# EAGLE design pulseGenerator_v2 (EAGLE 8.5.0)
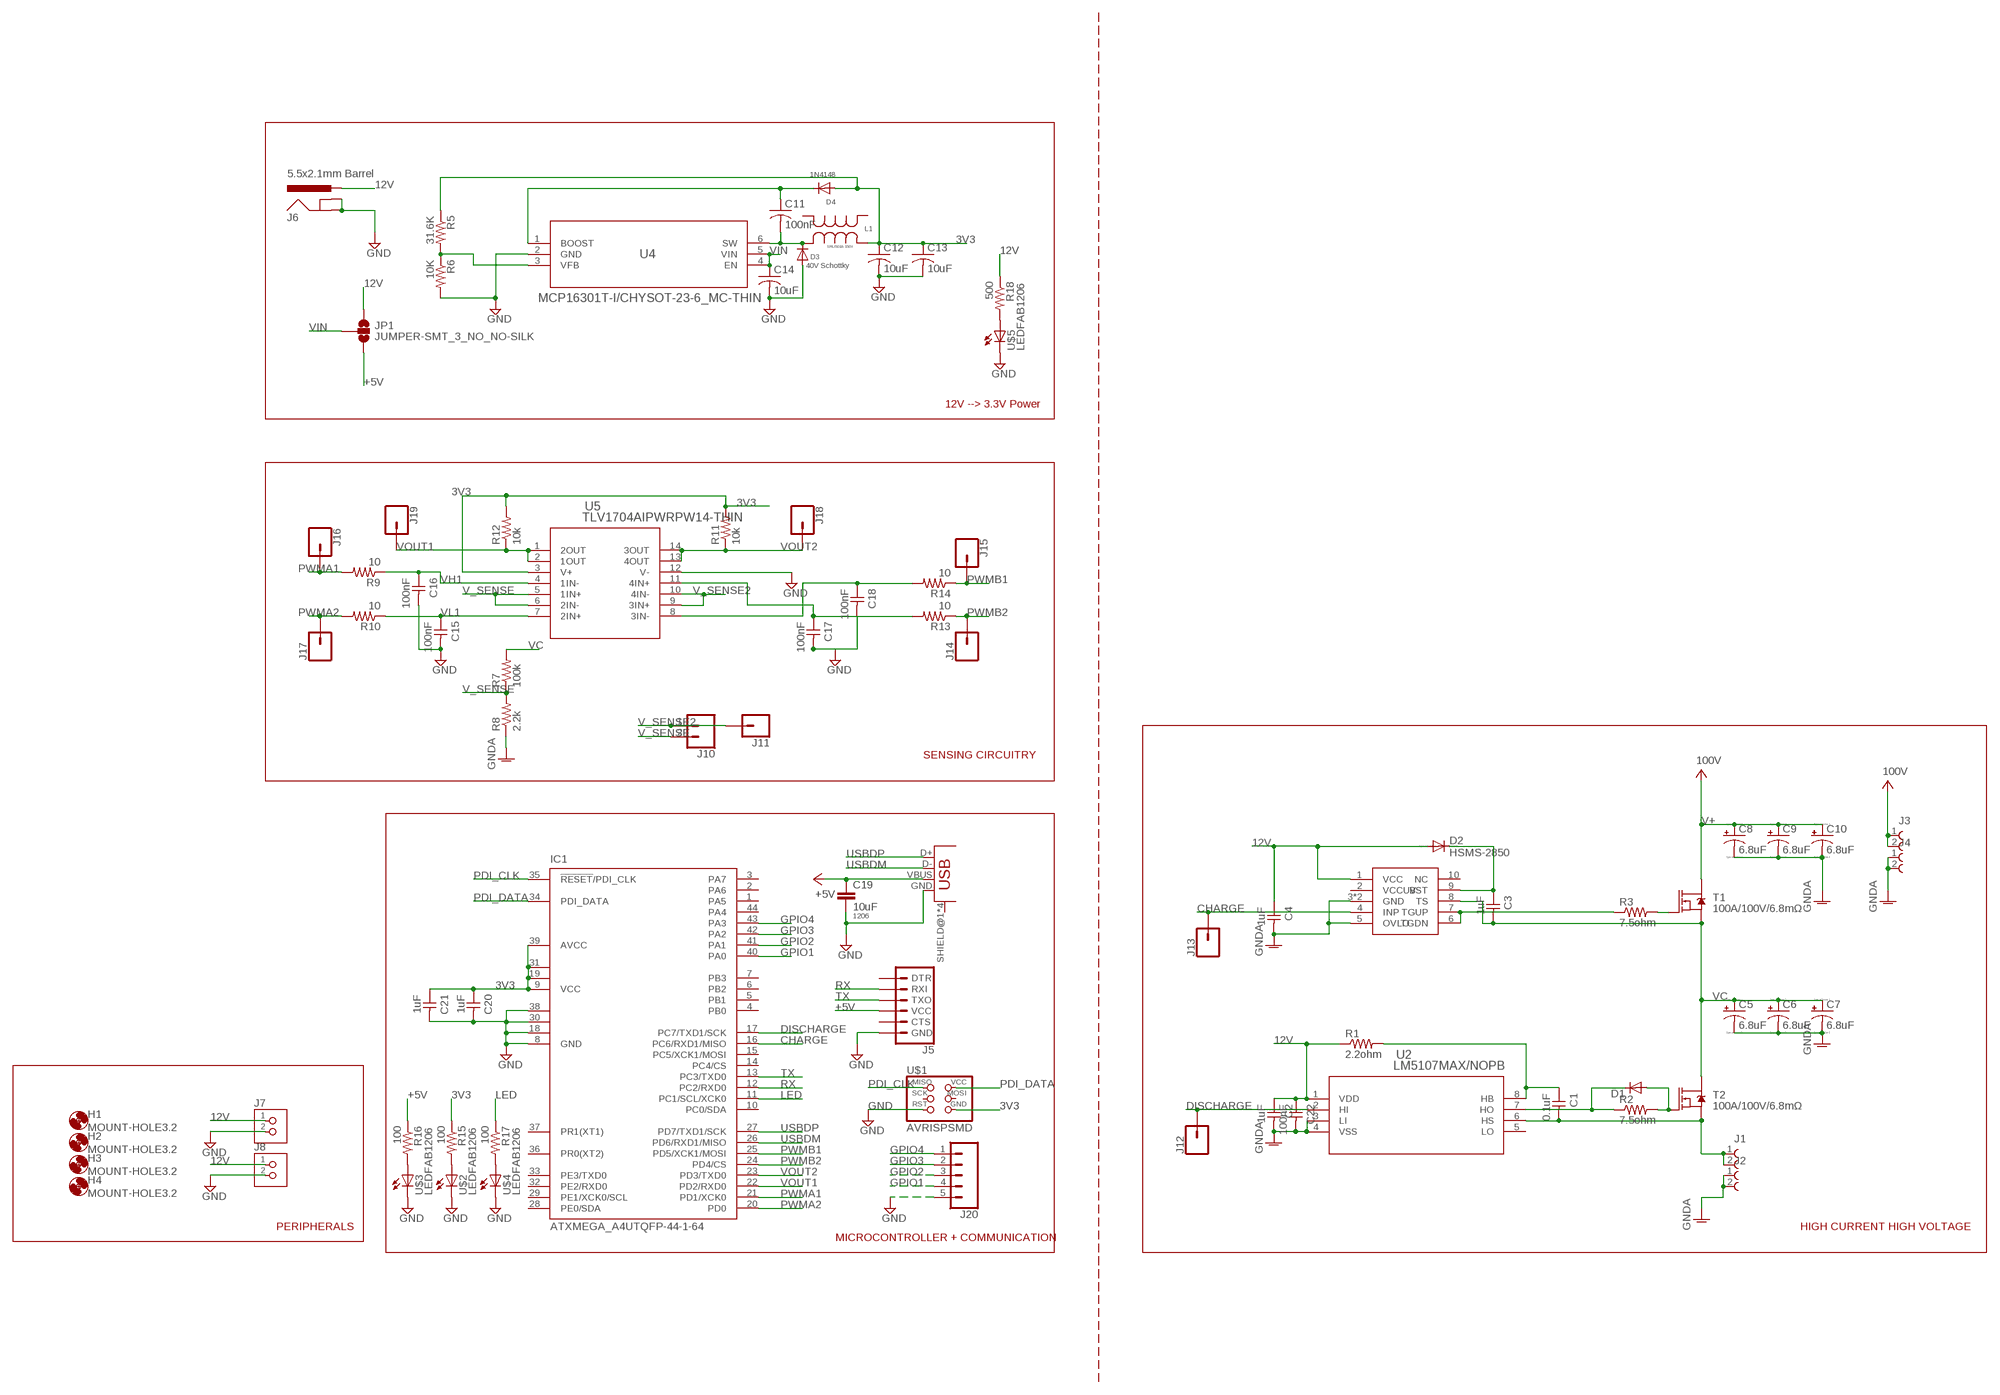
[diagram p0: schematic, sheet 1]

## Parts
C1  0.1uF  CAP-UNPOLARIZEDFAB  [C1206FAB]
C2  1uF  CAP-UNPOLARIZEDFAB  [C1206FAB]
C3  1uF  CAP-UNPOLARIZEDFAB  [C1206FAB]
C4  1uF  CAP-UNPOLARIZEDFAB  [C1206FAB]
C5  6.8uF  CPOL-USF  [PANASONIC_F]
C6  6.8uF  CPOL-USF  [PANASONIC_F]
C7  6.8uF  CPOL-USF  [PANASONIC_F]
C8  6.8uF  CPOL-USF  [PANASONIC_F]
C9  6.8uF  CPOL-USF  [PANASONIC_F]
C10  6.8uF  CPOL-USF  [PANASONIC_F]
C11  100nF  C-USC1206  [C1206]
C12  10uF  C-USC1206  [C1206]
C13  10uF  C-USC1206  [C1206]
C14  10uF  C-USC1206  [C1206]
C15  100nF  CAP-UNPOLARIZEDFAB  [C1206FAB]
C16  100nF  CAP-UNPOLARIZEDFAB  [C1206FAB]
C17  100nF  CAP-UNPOLARIZEDFAB  [C1206FAB]
C18  100nF  CAP-UNPOLARIZEDFAB  [C1206FAB]
C19  10uF  CAP1206  [1206]
C20  1uF  CAP-UNPOLARIZEDFAB  [C1206FAB]
C21  1uF  CAP-UNPOLARIZEDFAB  [C1206FAB]
C22  100nF  CAP-UNPOLARIZEDFAB  [C1206FAB]
D1  DIODESOD123  [SOD123]
D2  HSMS-2850  [SOT23]
D3  40V Schottky  DIODESOD-123  [SOD-123]
D4  1N4148  DIODESOD-123  [SOD-123]
H1  MOUNT-HOLE3.2  [3,2]
H2  MOUNT-HOLE3.2  [3,2]
H3  MOUNT-HOLE3.2  [3,2]
H4  MOUNT-HOLE3.2  [3,2]
IC1  ATXMEGA_A4UTQFP-44-1-64  [TQFP44-13THIN]
J1  691236510002  [691236510002]
J2  691236510002  [691236510002]
J3  691236510002  [691236510002]
J4  691236510002  [691236510002]
J5  6_PIN_SERIAL_TARGETRA_SMT  [6_PIN_SERIAL_TARGET_SIDE_RA_SMT]
J6  5.5x2.1mm Barrel  POWER_JACKSMD  [POWER_JACK_SMD]
J7  TERM-1X02-FABLAB  [ED555DS-2DS]
J8  TERM-1X02-FABLAB  [ED555DS-2DS]
J10  CONN_02  [1X02]
J11  CONN_01  [1X01]
J12  CONN_01  [1X01]
J13  CONN_01  [1X01]
J14  CONN_01  [1X01]
J15  CONN_01  [1X01]
J16  CONN_01  [1X01]
J17  CONN_01  [1X01]
J18  CONN_01  [1X01]
J19  CONN_01  [1X01]
J20  CONN_05  [1X05]
JP1  JUMPER-SMT_3_NO_NO-SILK  [SMT-JUMPER_3_NO_NO-SILK]
L1  SRU5018-150Y  [IND_BOURNS_SRU5018]
R1  2.2ohm  R-US_R1206  [R1206]
R2  7.5ohm  R-US_R1206  [R1206]
R3  7.5ohm  R-US_R1206  [R1206]
R5  31.6K  RES-US1206FAB  [R1206FAB]
R6  10K  R-US_R1206  [R1206]
R7  100k  R-US_R1206  [R1206]
R8  2.2k  R-US_R1206  [R1206]
R9  10  RES-US1206FAB  [R1206FAB]
R10  10  RES-US1206FAB  [R1206FAB]
R11  10k  RES-US1206FAB  [R1206FAB]
R12  10k  RES-US1206FAB  [R1206FAB]
R13  10  RES-US1206FAB  [R1206FAB]
R14  10  RES-US1206FAB  [R1206FAB]
R15  100  R-US_R1206  [R1206]
R16  100  R-US_R1206  [R1206]
R17  100  R-US_R1206  [R1206]
R18  500  R-US_R1206  [R1206]
T1  100A/100V/6.8mΩ  MOSFET-NCH-PSMN7R0  [TO-263/D2PAK]
T2  100A/100V/6.8mΩ  MOSFET-NCH-PSMN7R0  [TO-263/D2PAK]
U2  LM5107MAX/NOPB  [M08A]
U4  MCP16301T-I/CHYSOT-23-6_MC-THIN  [SOT-23-6_MC-THIN]
U5  TLV1704AIPWRPW14-THIN  [PW14_THIN]
U$1  AVRISPSMD  [2X03SMD]
U$2  LEDFAB1206  [LED1206FAB]
U$3  LEDFAB1206  [LED1206FAB]
U$4  LEDFAB1206  [LED1206FAB]
U$5  LEDFAB1206  [LED1206FAB]
U$6  LTC7001  [LTC7001-10MSOP]
X1  USB_MINIB  [USB_MINIB]

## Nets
3V3 [signal]: C12.1 C13.1 C20.1 C21.1 D4.A IC1.9(VCC) IC1.19(VCC1) IC1.31(VCC2) IC1.39(AVCC) L1.1 R5.1 R11.2 R12.2 R15.1 U5.3(V+) U$1.6(GND)
12V [signal]: C2.1 C4.1 C22.1 D2.1(A) J6.VIN0(PWR) J7.1 J8.1 JP1.1 R1.1 R18.1 U2.1(VDD) U$6.1(VCC)
+5V: C19.1 J5.4(VCC) JP1.3 R16.1 X1.VBUS
CHARGE [signal]: IC1.16(PC6/RXD1/MISO) J13.1 U$6.4(INP)
DISCHARGE [signal]: IC1.17(PC7/TXD1/SCK) J12.1 U2.2(HI)
GND: C12.2 C13.2 C14.2 C15.2 C16.2 C17.2 C18.2 C19.2 C20.2 C21.2 D3.A IC1.8(GND) IC1.18(GND1) IC1.30(GND2) IC1.38(GND3) J5.6(GND) J6.GND(GNDBREAK) J6.P$4(GND) J7.2 J8.2 J20.5 R6.2 U4.2(GND) U5.12(V-) U$1.5(RST) U$2.2(C) U$3.2(C) U$4.2(C) U$5.2(C) X1.GND
GNDA [POWER]: C2.2 C4.2 C5.- C6.- C7.- C8.- C9.- C10.- C22.2 J2.1 J2.2 J4.1 J4.2 R8.1 U2.3(LI) U2.4(VSS) U$6.3(GND) U$6.5(OVLO) U$6.P$1(GND)
GPIO1: IC1.40(PA0) J20.4
GPIO2: IC1.41(PA1) J20.3
GPIO3: IC1.42(PA2) J20.2
GPIO4: IC1.43(PA3) J20.1
LED [signal]: IC1.11(PC1/SCL/XCK0) R17.1
N$1 [signal]: C3.1 D2.3(C) U$6.9(BST)
N$2 [signal]: C1.1 R1.2 U2.8(HB)
N$3: R15.2 U$2.1(A)
N$4 [signal]: D1.ANODE(A) R2.2 T2.1(G)
N$5 [signal]: D1.CATHODE(C) R2.1 U2.7(HO)
N$6: R16.2 U$3.1(A)
N$9: R3.2 T1.1(G)
N$10 [signal]: R3.1 U$6.6(TGDN) U$6.7(TGUP)
N$11 [signal]: C17.1 R13.2 U5.11(4IN+)
N$12: R17.2 U$4.1(A)
N$13 [signal]: C11.2 D3.C L1.3 U4.6(SW)
N$14: R18.2 U$5.1(A)
N$15 [signal]: C11.1 D4.C U4.1(BOOST)
N$18 [signal]: C18.1 R14.2 U5.8(3IN-)
N$19 [signal]: R5.2 R6.1 U4.3(VFB)
OUTPUT [POWER]: C1.2 J1.1 J1.2 T2.3(S) U2.6(HS)
PDI_CLK [signal]: IC1.35(!RESET!/PDI_CLK) U$1.1(MISO)
PDI_DATA [signal]: IC1.34(PDI_DATA) U$1.2(VCC)
PWMA1 [signal]: IC1.21(PD1/XCK0) J16.1 R9.2
PWMA2 [signal]: IC1.20(PD0) J17.1 R10.2
PWMB1 [signal]: IC1.25(PD5/XCK1/MOSI) J15.1 R14.1
PWMB2 [signal]: IC1.24(PD4/CS) J14.1 R13.1
RX [signal]: IC1.12(PC2/RXD0) J5.3(RXI)
TX [signal]: IC1.13(PC3/TXD0) J5.2(TXO)
USBDM [signal]: IC1.26(PD6/RXD1/MISO) X1.D-
USBDP [signal]: IC1.27(PD7/TXD1/SCK) X1.D+
V+ [POWER]: C8.+ C9.+ C10.+ J3.1 J3.2 T1.2(D) ; supply symbol labelled 100V
V_SENSE [signal]: J10.2 R7.1 R8.2 U5.5(1IN+) U5.6(2IN-)
V_SENSE2 [signal]: J10.1 J11.1 U5.9(3IN+) U5.10(4IN-)
VC [signal]: C3.2 C5.+ C6.+ C7.+ R7.2 T1.3(S) T2.2(D) U$6.8(TS)
VH1 [signal]: C16.1 R9.1 U5.4(1IN-)
VIN: C14.1 JP1.2 U4.4(EN) U4.5(VIN)
VL1 [signal]: C15.1 R10.1 U5.7(2IN+)
VOUT1 [signal]: IC1.22(PD2/RXD0) J19.1 R12.1 U5.1(2OUT) U5.2(1OUT)
VOUT2 [signal]: IC1.23(PD3/TXD0) J18.1 R11.1 U5.13(4OUT) U5.14(3OUT)
Unconnected: IC1.1(PA5) IC1.2(PA6) IC1.3(PA7) IC1.4(PB0) IC1.5(PB1) IC1.6(PB2) IC1.7(PB3) IC1.10(PC0/SDA) IC1.14(PC4/CS) IC1.15(PC5/XCK1/MOSI) IC1.28(PE0/SDA) IC1.29(PE1/XCK0/SCL) IC1.32(PE2/RXD0) IC1.33(PE3/TXD0) IC1.36(PR0(XT2)) IC1.37(PR1(XT1)) IC1.44(PA4) J5.1(DTR) J5.5(CTS) L1.2 L1.4 U2.5(LO) U$1.3(SCK) U$1.4(MOSI) U$6.2(VCCUV) U$6.10(NC) X1.SHIELD@1(SHIELD) X1.SHIELD@2(SHIELD) X1.SHIELD@3(SHIELD) X1.SHIELD@4(SHIELD)

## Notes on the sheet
- 12V --> 3.3V Power
- SENSING CIRCUITRY
- PERIPHERALS | HIGH CURRENT HIGH VOLTAGE
- MICROCONTROLLER + COMMUNICATION

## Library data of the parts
C1-C4 C15-C18 C20-C22 = fab:CAP-UNPOLARIZED
C5-C10 = resistor:CPOL-US: POLARIZED CAPACITOR, American symbol
C11-C14 = resistor:C-US: CAPACITOR, American symbol
C19 = borkedlabs-passives:CAP: Capacitor; PACKAGE: 1206
D1 = fab:DIODE: DIODE
D2 = avago:HSMS-2850: Surface Mount Microwave Schottky Detector Diodes
D3 D4 = adafruit:DIODE: Diode
H1-H4 = holes:MOUNT-HOLE: MOUNTING HOLE with drill center marker
IC1 = fab:ATXMEGA_A4U
J1-J4 = Wurth_Elektronik_Electromechanic_Terminal_Blocks_Connectors_rev17a:691236510002
J5 = SparkFun-Connectors:6_PIN_SERIAL_TARGET: 6-pin header connection for use with the "FTDI BASIC" pinout - TARGET SIDE. Also known as "Arduino Serial Program Header". It is used to mate with our FTDI Basic serial programmers using the Arduino IDE. Note, this device has "TARGET" in the name. It is intended to be used on a design that contains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; PROD_ID: CONN-08971
J6 = SparkFun-Connectors:POWER_JACK: Power Jack Connector This is the standard 5.5mm barrel jack for power. The PTH is the most common, proven, reliable, footprint. The Slot footprint only works if the mill layer is transmitted to the PCB fab house so be warned. Here are the connectors we sell at SparkFun: DC Barrel Power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; PROD_ID: CONN-08106; SF_ID: PRT-12748
J7 J8 = fab:TERM-1X02: 3.5mm terminal block, 2 positions ED555-2DS as found in the fablab inventory.
J10 = SparkFun-Connectors:CONN_02: Multi connection point. Often used as Generic Header-pin footprint for 0.1 inch spaced/style header connections
J11-J19 = SparkFun-Connectors:CONN_01: Single connection point. Often used as Generic Header-pin footprint for 0.1 inch spaced/style header connections
J20 = SparkFun-Connectors:CONN_05: Multi connection point. Often used as Generic Header-pin footprint for 0.1 inch spaced/style header connections On any of the 0.1 inch spaced packages, you can populate with these: Break Away Headers - Straight (PRT-00116) Break Away Male Headers - Right Angle (PRT-00553) Female Headers (PRT-00115)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
JP1 = SparkFun-Jumpers:JUMPER-SMT_3_NO: Normally open jumper This jumper has three pads in close proximity to each other. Apply solder to close the connection(s).
L1 = will:SRU5018-150Y; MANUFACTURER_PART_NUMBER: SRU5018150Y; VENDOR: Bourns Electronics
R1-R3 R6-R8 R15-R18 = resistor:R-US_: RESISTOR, American symbol
R5 R9-R14 = fab:RES-US: Resistor (US Symbol)
T1 T2 = SparkFun-DiscreteSemi:MOSFET-NCH: N-channel MOSFETs Voltage controlled devices that allow control of high current outputs. SparkFun Products: SparkFun OpenScale SparkFun Digital Sandbox SparkFun Monster Moto Shield SparkFun MOSFET Power Controller; PROD_ID: TRANS-12437
U2 = lm5107_half_bridge_gate_driver:LM5107MAX/NOPB; MANUFACTURER_PART_NUMBER: LM5107MAXNOPB; VENDOR: Texas Instruments
U4 = will:MCP16301T-I/CHY
U5 = will:TLV1704AIPWR
U$1 = fab:AVRISP
U$2-U$5 = fab:LED: LED
U$6 = will:LTC7001
X1 = fab:USB_MINIB

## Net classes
0 default: width 0.305 mm, clearance 0.45 mm
1 POWER: width 1.27 mm, clearance 2 mm
2 signal: width 0.25 mm, clearance 0.2 mm

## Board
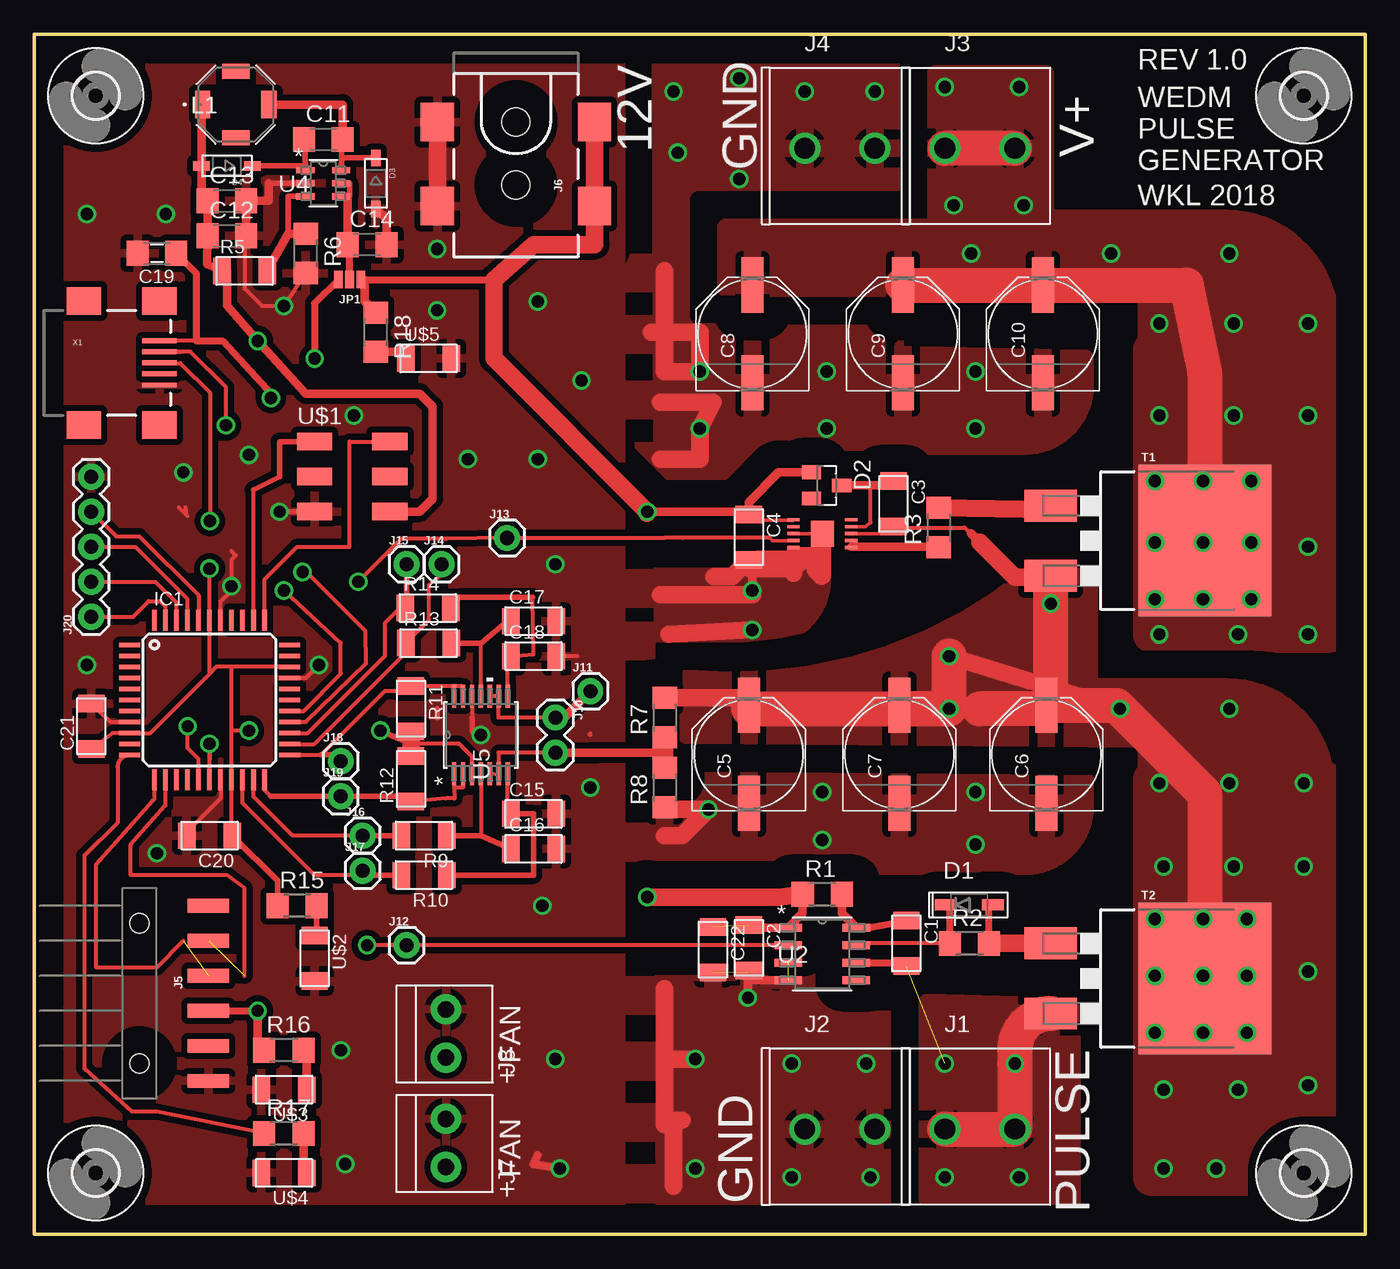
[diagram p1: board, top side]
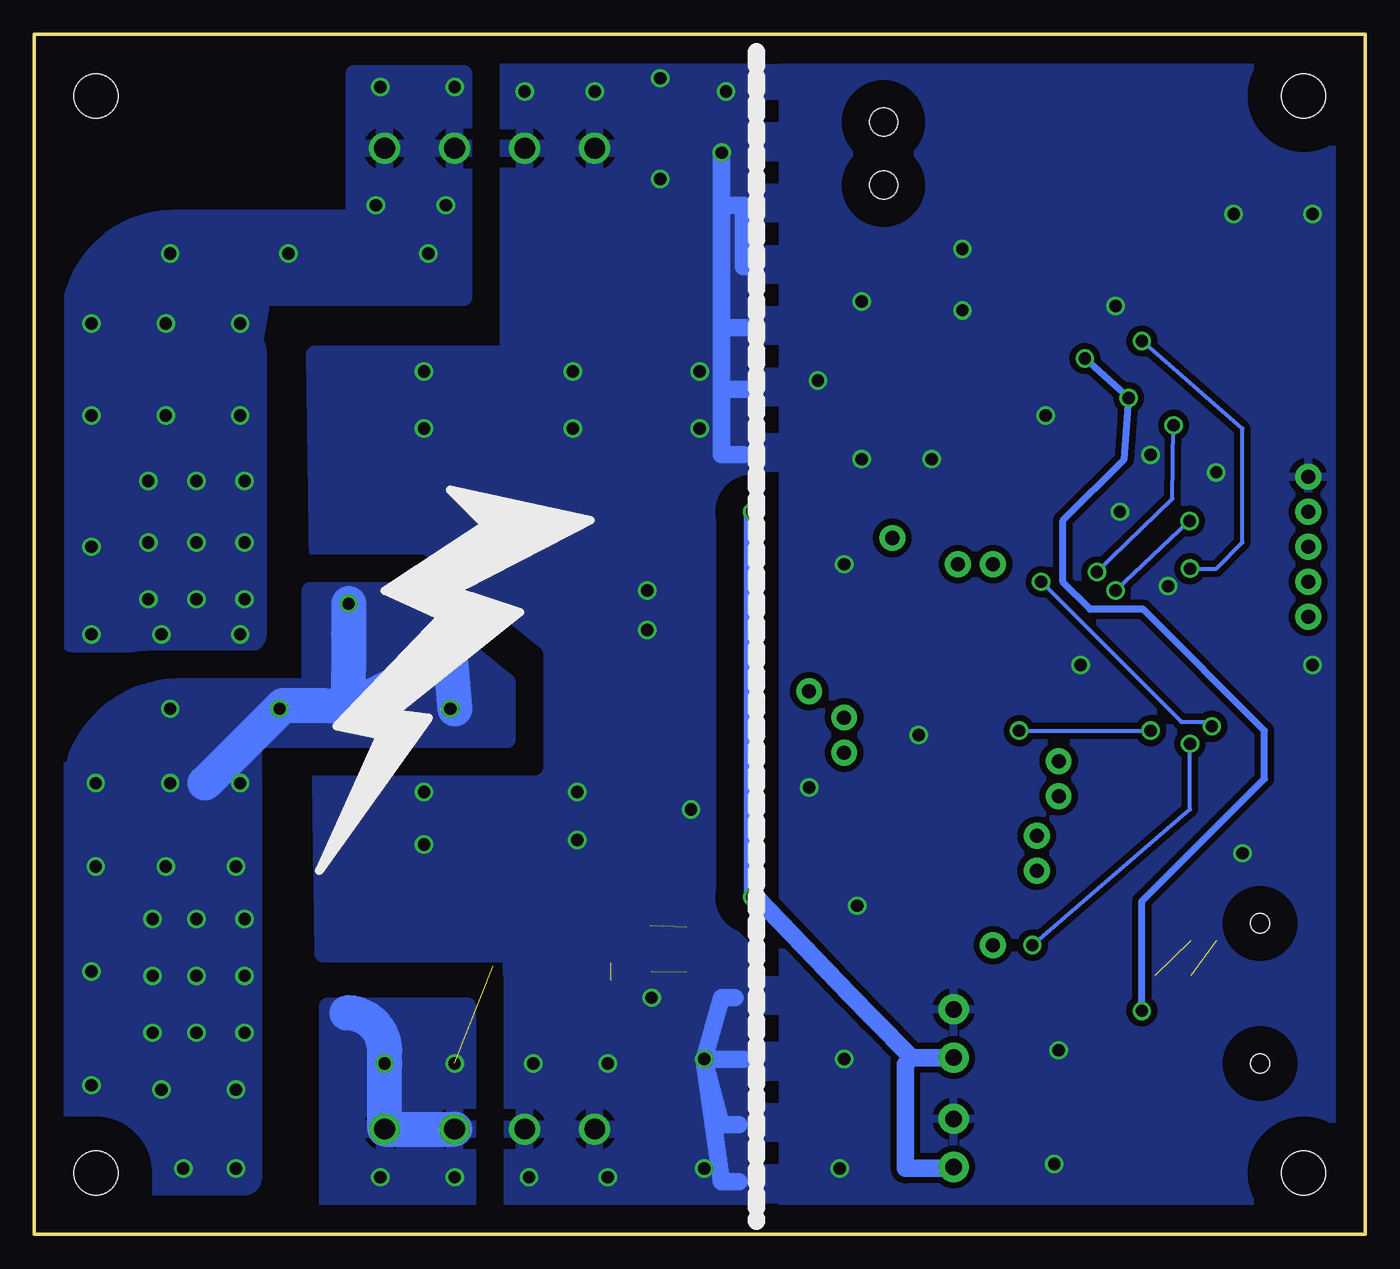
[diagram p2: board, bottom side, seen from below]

Size 96.52 x 87 mm. Coordinates in mm from the lower left corner, seen from the top.
Outline: 0,0 96.52,0 96.52,87 0,87 0,0
Copper layers (1*16): Top 0.035mm / dielectric 1.5mm / Bottom 0.035mm
Design rules "default *": minimum track width 6mil, minimum drill 0.35mm, track to track 0.2mm, track to pad 0.2mm, pad to pad 0.2mm, via to via 0.2mm, smd to smd 0mil, copper to edge 2mm, drill to drill 6mil, minimum pad ring 10mil, minimum via ring 8mil, stop-mask expansion 4mil, vias tented up to drill 0mil, thermal gap 0.45mm

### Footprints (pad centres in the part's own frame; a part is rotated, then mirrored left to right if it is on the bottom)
C1206FAB = smd 1.27 x 1.905: 1 -1.651,0; 2 1.651,0
PANASONIC_F = smd 4 x 1.6: + 3.55,0; - -3.55,0
C1206 = smd 1.6 x 1.8: 1 -1.4,0; 2 1.4,0
1206 = smd 1.6 x 1.8: 1 -1.4,0; 2 1.4,0
SOD123 = smd 1.6 x 0.8: ANODE 1.7,0; CATHODE -1.7,0
SOT23 = smd 1 x 1.4: 1 -0.95,-1.1; 2 0.95,-1.1; 3 0,1.1
SOD-123 = smd 1.2 x 0.7: A 1.85,0; C -1.85,0
3,2 = hole 3.2: 0,0
TQFP44-13THIN = smd 1.524 x 0.33: 1 -5.8,4; 2 -5.8,3.2; 3 -5.8,2.4; 4 -5.8,1.6; 5 -5.8,0.8; 6 -5.8,0; 7 -5.8,-0.8; 8 -5.8,-1.6; 9 -5.8,-2.4; 10 -5.8,-3.2; 11 -5.8,-4; 23 5.8,-4; 24 5.8,-3.2; 25 5.8,-2.4; 26 5.8,-1.6; 27 5.8,-0.8; 28 5.8,0; 29 5.8,0.8; 30 5.8,1.6; 31 5.8,2.4; 32 5.8,3.2; 33 5.8,4 | smd 0.33 x 1.524: 12 -4,-5.8; 13 -3.2,-5.8; 14 -2.4,-5.8; 15 -1.6,-5.8; 16 -0.8,-5.8; 17 0,-5.8; 18 0.8,-5.8; 19 1.6,-5.8; 20 2.4,-5.8; 21 3.2,-5.8; 22 4,-5.8; 34 4,5.8; 35 3.2,5.8; 36 2.4,5.8; 37 1.6,5.8; 38 0.8,5.8; 39 0,5.8; 40 -0.8,5.8; 41 -1.6,5.8; 42 -2.4,5.8; 43 -3.2,5.8; 44 -4,5.8
691236510002 = drill 1.5: 1 -2.54,0; 2 2.54,0
6_PIN_SERIAL_TARGET_SIDE_RA_SMT = smd 1 x 3: 1 -6.35,5; 2 -3.81,5; 3 -1.27,5; 4 1.27,5; 5 3.81,5; 6 6.35,5 | hole 1.4: -5.08,0; 5.08,0
POWER_JACK_SMD = smd 2.8 x 2.4: GND 0,-5.7; P$4 6.1,-5.7; VIN0 0,5.7; VIN1 6.1,5.7 | hole 2.032: 0,0; 4.572,0
ED555DS-2DS = drill 1.2 pad 2.184: 1 1.8,0; 2 -1.7,0
1X02 = drill 1.016 pad 1.88: 1 0,0; 2 2.54,0
1X01 = drill 1.016 pad 1.88: 1 0,0
1X05 = drill 1.016 pad 1.88: 1 0,0; 2 2.54,0; 3 5.08,0; 4 7.62,0; 5 10.16,0
SMT-JUMPER_3_NO_NO-SILK = smd 0.635 x 1.27: 1 -0.813,0; 2 0,0; 3 0.813,0
IND_BOURNS_SRU5018 = smd 1.092 x 2.007: 1 -2.4,0; 3 2.4,0 | smd 2.007 x 1.092: 2 0,-2.4; 4 0,2.4
R1206 = smd 1.6 x 1.803: 1 -1.422,0; 2 1.422,0
R1206FAB = smd 1.27 x 1.905: 1 -1.651,0; 2 1.651,0
TO-263/D2PAK = smd 2.32 x 3.81: 1 -2.54,-7.045; 3 2.54,-7.045 | smd 11 x 9.65: 2 0,4.125
M08A = smd 1.981 x 0.559: 1 -2.464,1.905; 2 -2.464,0.635; 3 -2.464,-0.635; 4 -2.464,-1.905; 5 2.464,-1.905; 6 2.464,-0.635; 7 2.464,0.635; 8 2.464,1.905
SOT-23-6_MC-THIN = smd 1.321 x 0.457: 1 -1.295,0.95; 2 -1.295,0; 3 -1.295,-0.95; 4 1.295,-0.95; 5 1.295,0; 6 1.295,0.95
PW14_THIN = smd 1.676 x 0.305: 1 -2.819,1.95; 2 -2.819,1.3; 3 -2.819,0.65; 4 -2.819,0; 5 -2.819,-0.65; 6 -2.819,-1.3; 7 -2.819,-1.95; 8 2.819,-1.95; 9 2.819,-1.3; 10 2.819,-0.65; 11 2.819,0; 12 2.819,0.65; 13 2.819,1.3; 14 2.819,1.95
2X03SMD = smd 2.54 x 1.27: 1 -2.54,2.54; 2 2.92,2.54; 3 -2.54,0; 4 2.92,0; 5 -2.54,-2.54; 6 2.92,-2.54
LED1206FAB = smd 1.27 x 1.905: 1 -1.651,0; 2 1.651,0
LTC7001-10MSOP = smd 0.24 x 0.889: 1 -1,-2.1; 2 -0.5,-2.1; 3 0,-2.1; 4 0.5,-2.1; 5 1,-2.1; 6 1,2.1; 7 0.5,2.1; 8 0,2.1; 9 -0.5,2.1; 10 -1,2.1 | smd 1.88 x 1.68: P$1 0,0
USB_MINIB = smd 2.5 x 0.35: D+ 3.77,0; D- 3.77,0.8; GND 3.77,-1.6; ID 3.77,-0.8; VBUS 3.77,1.6 | smd 2.5 x 2: SHIELD@1 -1.73,-4.5; SHIELD@2 -1.73,4.5; SHIELD@3 3.77,4.5; SHIELD@4 3.77,-4.5

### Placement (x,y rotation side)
C1  63.25,21.08 270 top
C2  51.82,20.76 270 top
C3  62.32,52.96 270 top
C4  51.82,50.55 270 top
C5  51.82,34.8 90 top
C6  73.41,34.8 90 top
C7  62.74,34.8 90 top
C8  52.07,65.28 90 top
C9  62.99,65.28 90 top
C10  73.15,65.28 90 top
C11  20.95,79.38 0 top
C12  13.97,72.39 0 top
C13  13.97,74.93 0 top
C14  24.13,71.75 0 top
C15  36.2,30.48 0 top
C16  36.2,27.94 0 top
C17  36.2,44.45 0 top
C18  36.2,41.91 0 top
C19  8.89,71.12 180 top
C20  12.7,28.89 180 top
C21  4.13,36.83 90 top
C22  49.21,20.64 270 top
D1  67.82,23.88 0 top
D2  57.47,54.29 270 top
D3  24.77,76.2 270 top
D4  13.97,77.47 180 top
H1  4.45,4.45 0 top
H2  92.08,82.55 0 top
H3  4.45,82.55 0 top
H4  92.08,4.45 0 top
IC1  12.7,38.73 0 top
J1  68.58,7.62 0 top
J2  58.42,7.62 0 top
J3  68.58,78.74 0 top
J4  58.42,78.74 0 top
J5  7.62,17.46 270 top
J6  34.92,80.64 270 top
J7  29.84,6.67 270 top
J8  29.84,14.61 270 top
J10  37.78,37.47 270 top
J11  40.32,39.37 0 top
J12  26.99,20.95 0 top
J13  34.29,50.48 0 top
J14  29.53,48.58 0 top
J15  26.99,48.58 0 top
J16  23.81,28.89 0 top
J17  23.81,26.35 0 top
J18  22.23,34.29 0 top
J19  22.23,31.75 0 top
J20  4.13,44.77 90 top
JP1  22.86,69.22 180 top
L1  14.61,81.92 0 top
R1  57.15,24.64 0 top
R2  67.82,21.08 0 top
R3  65.6,51.24 90 top
R5  15.24,69.85 0 top
R6  19.68,71.12 270 top
R7  45.72,37.47 90 top
R8  45.72,32.38 90 top
R9  28.26,28.89 180 top
R10  28.26,26.04 180 top
R11  27.3,38.1 270 top
R12  27.3,33.02 90 top
R13  28.57,42.86 0 top
R14  28.55,45.4 0 top
R15  19.05,23.81 0 top
R16  18.1,13.34 0 top
R17  18.1,7.3 0 top
R18  24.77,65.41 270 top
T1  80.77,50.29 270 top
T2  80.77,18.54 270 top
U2  57.15,20.32 0 top
U4  20.95,76.2 0 top
U5  32.38,36.2 90 top
U$1  22.86,54.93 0 top
U$2  20.32,20 270 top
U$3  18.1,10.48 180 top
U$4  18.1,4.45 180 top
U$5  28.57,63.5 0 top
U$6  57.15,50.8 270 top
X1  5.31,63.18 0 top

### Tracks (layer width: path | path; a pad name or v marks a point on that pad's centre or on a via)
3V3  (via drill 0.89)
  Top 0.305: 31.75,33.31 arc90 U5.3 31.73,34.61 30.79,35.56 27.3,35.56 | IC1.19 14.3,29.09 C20.1 | IC1.19 | C21.1 5.67,36.34 IC1.9 8.39,36.34 12.7,40.64 | 12.7,40.64 IC1.39 v12.7,48.26 | IC1.31 14.29,41.13 | 14.29,41.13 13.2,41.13 12.7,40.64 | 14.29,36.51 14.29,32.95 IC1.19 | 14.29,36.51 14.29,41.13 | v15.56,36.51 14.29,36.51 | IC1.19
  Top 0.406: 27.3,35.56 v25.08,36.51 | R15.1 17.63,25.61 C20.1
  Top 0.61: 12.12,82.55 D4.A 12.12,74.93 C13.1 C12.1 12.54,70.33 R5.1 13.97,69.85 13.97,67.31 v16.19,64.77 19.68,60.96 27.94,60.96 28.89,60.01 28.89,53.34 27.94,52.39 U$1.6 | 12.12,82.55 12.06,81.92 | 12.12,82.55 12.21,82.55 L1.1
  Top 1.27: R12.2 27.3,35.56 R11.2
  Bottom 0.305: v25.08,36.51 v15.56,36.51 | v12.7,48.26 10.79,48.26 8.89,50.16 8.89,58.42 v16.19,64.77
12V  (via drill 0.89)  (1 unrouted)
  Top 0.241: U$6.1 55.05,51.75 51.82,51.75 C4.1
  Top 0.508: JP1.1 23.93,69.22 33.34,69.22
  Top 0.61: R1.1 55.73,23.27 U2.1 52.07,22.23 C2.1 | R18.1 23.93,67.66 23.93,69.22 | D2.1 53.97,55.24 51.82,53.09 C4.1 51.63,52.39 v44.45,52.39
  Top 1.27: J6.VIN0 40.64,80.63 40.64,71.75 36.2,71.75 33.34,69.22 33.34,63.5 v44.45,52.39 44.45,52.26 | R1.1 54.01,24.45 v44.45,24.45
  Bottom 1.27: v44.45,52.39 v44.45,24.45 44.13,24.45 37.31,17.31 35.79,15.72 32.87,12.8 | J8.1 32.87,12.8 | J7.1 29.95,4.76 33.34,4.76 33.34,12.34 32.87,12.8
+5V  (via drill 0.89)
  Top 0.305: X1.VBUS 9.84,64.78 | 9.84,64.78 10.3,64.78 | 11.75,64.77 11.73,64.78 9.84,64.78
  Top 0.508: JP1.3 20.32,67.49 v20.32,63.5 | C19.1 11.75,69.66 11.75,64.77 13.65,64.77 17.27,60.83 v17.14,60.64 | J5.4 v16.19,16.19
  Top 0.61: R16.1 arc-90 16.19,13.82 v16.19,16.19
  Bottom 0.508: v20.32,63.5 v17.14,60.64 17.46,56.2 21.91,51.75 21.91,47.27 19.93,45.3 16.09,45.3 7.3,36.51 7.3,33.02 16.19,24.13 v16.19,16.19
CHARGE  (via drill 0.89)
  Top 0.241: U$6.4 53.52,50.3 53.34,50.48
  Top 0.305: v11.11,36.83 11.11,35.24 11.9,34.45 IC1.16 | v23.5,47.31 26.61,50.42 29.84,50.42 J13.1 45.72,50.48 46.99,50.48 53.34,50.48
  Bottom 0.305: v23.5,47.31 13.34,37.15 11.43,37.15 v11.11,36.83
DISCHARGE  (via drill 0.89)
  Top 0.305: U2.2 v24.13,20.95 J12.1 | 12.7,34.41 v12.7,35.56 IC1.17
  Bottom 0.305: v24.13,20.95 12.7,30.8 v12.7,35.56
GND  (via drill 0.89)
  Top 0.305: C12.2 arc90 15.24,72.26 15.24,68.58 16.51,67.31 v18.1,67.31 R6.2 | U5.12 31.75,39.06 31.75,37.47 | IC1.18 13.5,31.6 11.3,29.4 C20.2 | IC1.8 5.54,37.13 C21.2 | 10.49,52.69 10.95,52.23 | 10.95,52.23 11.11,52.07 | IC1.30 19.7,40.34 v20.64,41.27 | 40.31,36.2 40.31,36.31 | 39.37,41.91 C18.2 | IC1.38 13.5,45.88 14.29,46.67 14.29,48.9 14.61,49.21 14.29,49.53 | 10.95,52.69 10.95,52.23
  Top 0.406: U4.2 16.99,76.2 | 31.75,37.47 31.75,36.83 arc90 32.11,36.2 | 29.21,37.47 29.21,38.1 | U$1.5 v17.78,52.39
  Top 0.61: 16.99,76.2 16.99,74.93 C13.2 C12.2 | 29.23,74.3 29.21,74.3 | C14.2 25.53,73.58 D3.A | 36.51,5.71 36.2,5.08 v38.1,4.76
  Top 1.27: J6.GND 29.23,74.3
  other vias: 29.21,71.44 39.69,61.91 3.81,41.27 8.89,27.62 36.51,56.2 14.29,46.99 40.32,32.38 3.81,73.98 9.53,73.98 36.83,23.81 37.78,12.7 22.23,13.34 22.54,5.08 37.78,48.58 36.51,67.63 29.21,66.99 31.43,56.2 32.38,36.2 23.18,59.37 10.79,55.24 15.56,56.52
  pour Top (rank 2): 0.32,0 42.55,0 42.55,87 0.32,87
  pour Bottom (rank 2): 42.23,1.59 42.23,88.27 0,87 0,0
GNDA  (via drill 0.89)  (2 unrouted)
  Top 0.241: U$6.P$1 U$6.3 | C4.2 55.05,48.96 U$6.5 55.05,49.21 | 55.05,47.94 55.05,47.62 55.24,47.62
  Top 0.61: C4.2 51.82,47.88 52.07,47.88 v52.07,46.67 | v51.75,17.14 51.75,18.41 | 51.75,18.41 51.75,19.05 C2.2 | U2.4 51.75,18.41
  Top 1.27: R8.1 arc90 45.89,30.8 v48.9,30.8 46.99,28.89 45.72,28.89 | 46.35,8.26 46.35,3.49 | 45.72,12.7 45.72,17.78 | v47.94,12.7 45.72,12.7 | 45.72,12.7 45.72,8.26 | 45.72,7.94 45.72,8.26 | 45.72,8.26 46.35,8.26 | 46.35,8.26 46.99,8.26 | v52.07,43.81 46.04,43.5 | v52.07,46.67 52.07,46.35 45.4,46.35 | 45.4,56.2 48.26,56.2 v48.26,58.42 49.21,60.33 45.4,60.33 | 44.77,65.41 48.26,65.41 v48.26,62.55 45.72,62.55 45.72,69.85 | 55.05,47.94 55.05,48.26 | 55.05,48.26 55.05,49.21 56.83,49.21 57.15,49.53 | C4.2 52.49,48.93 54.97,48.93 | C4.2 52.45,48.26 55.05,48.26 | C4.2 50.6,47.68 49.3,47.68 | U$6.P$1 57.15,49.53 | 57.15,49.53 57.15,47.75 57.1,47.7 56.67,48.13 56.67,48.84 55.63,48.84 55.05,48.26
  Bottom 1.27: v47.94,12.7 46.67,17.14 45.72,17.14 | v47.94,12.7 45.09,12.7 | v47.94,12.7 46.67,7.94 45.4,7.94 | v47.94,12.7 46.67,3.81 45.4,3.81 | v46.67,78.42 46.67,74.61 45.09,74.61 45.09,70.17 44.77,70.17 | v46.67,78.42 46.67,65.72 44.77,65.72 | v46.67,78.42 46.67,61.28 44.77,61.28 | v46.67,78.42 46.67,56.52 45.09,56.52
  other vias: 51.12,76.52 46.35,82.87 57.47,62.55 68.26,62.55 68.26,58.42 68.26,28.26 57.15,32.07 68.26,32.07 54.93,12.38 60.33,12.38 57.15,28.57 51.12,83.82 57.47,58.42 47.94,4.76 55.88,82.87 54.93,4.13 60.64,4.13 60.96,82.87
  pour Top (rank 2): 61.91,0 61.91,17.78 57.15,17.78 57.15,26.67 71.86,26.67 arc90 76.2,31.01 76.2,33.02 48.26,33.02 48.26,38.84 arc-90 52.6,43.18 52.81,43.18 arc90 57.15,47.52 57.15,57.15 71.86,57.15 arc90 76.2,61.49 76.2,63.5 62.44,63.82 62.55,87 45.4,87 45.72,0
  pour Bottom (rank 2): 61.91,0.32 61.91,20.32 75.56,20.32 76.2,63.82 62.12,63.82 62.23,76.52 62.23,87 45.09,87 45.4,0.32
  pour Top (rank 2): 40.32,4.76 40.01,2.54 46.35,2.54 46.35,4.76
  pour Top (rank 2): 40.32,9.21 40.01,6.99 46.35,6.99 46.35,9.21
  pour Top (rank 2): 40.32,13.65 40.01,11.43 46.35,11.43 46.35,13.65
  pour Top (rank 2): 40.32,18.41 40.01,16.19 46.35,16.19 46.35,18.41
  pour Top (rank 2): 41.27,47.94 40.96,45.72 47.31,45.72 47.31,47.94
  pour Top (rank 2): 41.27,44.13 40.96,41.91 47.31,41.91 47.31,44.13
  pour Top (rank 2): 39.69,66.36 39.37,64.14 45.72,64.14 45.72,66.36
  pour Top (rank 2): 39.69,61.59 39.37,59.37 45.72,59.37 45.72,61.59
  pour Top (rank 2): 39.69,57.15 39.37,54.93 45.72,54.93 45.72,57.15
  pour Bottom (rank 2): 40.32,4.76 40.01,2.54 46.35,2.54 46.35,4.76
  pour Bottom (rank 2): 40.64,9.21 40.32,6.99 46.67,6.99 46.67,9.21
  pour Bottom (rank 2): 40.64,13.65 40.32,11.43 46.67,11.43 46.67,13.65
  pour Bottom (rank 2): 40.32,18.41 40.01,16.19 46.35,16.19 46.35,18.41
  pour Bottom (rank 2): 40.96,57.78 40.64,55.56 46.99,55.56 46.99,57.78
  pour Bottom (rank 2): 40.96,62.55 40.64,60.33 46.99,60.33 46.99,62.55
  pour Bottom (rank 2): 40.64,66.99 40.32,64.77 46.67,64.77 46.67,66.99
  pour Bottom (rank 2): 40.64,71.44 40.32,69.22 46.67,69.22 46.67,71.44
  pour Bottom (rank 2): 40.64,75.88 40.32,73.66 46.67,73.66 46.67,75.88
  pour Bottom (rank 2): 40.64,80.33 40.32,78.11 46.67,78.11 46.67,80.33
  pour Bottom (rank 2): 40.64,84.77 40.32,82.55 46.67,82.55 46.67,84.77
  pour Top (rank 2): 39.69,70.8 39.37,68.58 45.72,68.58 45.72,70.8
  pour Top (rank 2): 41.59,29.53 41.27,27.3 47.62,27.3 47.62,29.53
GPIO1
  Top 0.305: J20.4 5.91,50.6 7.61,50.6 11.9,46.32 IC1.40
GPIO2
  Top 0.305: IC1.41 11.07,44.57 11.07,46.08 7.3,49.85 J20.3
GPIO3
  Top 0.305: IC1.42 10.27,44.57 10.27,45.81 8.77,47.31 J20.2
GPIO4
  Top 0.305: IC1.43 9.47,44.57 9.47,45.55 9.12,45.9 8.29,45.9 7.15,44.77 J20.1
LED
  Top 0.305: IC1.11 arc90 6.03,33.87 6.03,29.84 3.62,27.43 3.62,12.03 7.08,8.89 8.89,8.89 R17.1
N$1
  Top 0.241: U$6.9 60.27,51.3 60.64,51.62
  Top 0.254: 62.32,54.29 C3.1
  Top 0.305: 60.64,51.62 60.64,54.29
  Top 0.61: D2.3 60.64,54.29 62.32,54.29
N$2
  Top 0.508: U2.8 60.45,22.23 C1.1
  Top 0.61: R1.2 58.57,23.27 U2.8
N$3
  Top 0.406: R15.2 20.47,21.8 U$2.1
N$4
  Top 0.508: R2.2 69.24,23.6 D1.ANODE
  Top 1.27: R2.2 T2.1
N$5
  Top 0.305: R2.1 59.74,21.08 U2.7
  Top 0.508: R2.1 66.4,23.6 D1.CATHODE
N$6
  Top 0.61: U$3.1 19.75,13.11 R16.2
N$9
  Top 1.27: 73.47,52.58 arc90 T1.1 73.73,52.51 R3.2
N$10  (1 unrouted)
  Top 0.241: U$6.7 59.25,49.85
  Top 0.305: R3.1 65.11,49.82 65.09,49.85
  Top 0.61: 65.09,49.85 59.25,49.85
N$11
  Top 0.305: U5.11 32.38,42.86
  Top 0.406: C17.1 34.29,44.45 32.38,42.86 R13.2
N$12
  Top 0.61: U$4.1 19.52,4.67 R17.2
N$13
  Top 0.406: 22.3,79.38 U4.6 22.3,78.05 D3.C
  Top 0.61: 22.3,79.38 C11.2 22.36,81.92 L1.3
N$14
  Top 0.61: U$5.1 26.44,63.98 R18.2
N$15
  Top 0.406: 19.61,79.38 U4.1 arc90 19.29,77.47 D4.C
  Top 0.61: 19.61,79.38 C11.1
N$18
  Top 0.305: U5.8 34.34,41.91 | C18.1 36.2,42.04 36.14,46.19
  Top 0.406: 34.34,41.91 C18.1 | 36.14,46.19 30.73,46.18 30.2,45.64 R14.2
N$19
  Top 0.406: U4.3 18.41,75.25 18.41,72.54
  Top 0.61: R6.1 18.41,72.54 R5.2
OUTPUT  (via drill 0.89)  (1 unrouted)
  Top 0.508: U2.6 63.24,19.68 C1.2
  Top 2.54: T2.3 arc90 71.12,13.39 v71.12,12.38 J1.2 J1.1
  Bottom 2.54: 73.86,16.05 arc90 71.12,13.31 v71.12,12.38 J1.2 J1.1
  other vias: 66.04,12.38 66.04,4.13 71.44,4.13
  pour Top: 64.77,16.83 75.25,16.51 75.25,2.22 64.77,2.54
  pour Bottom: 65.09,16.51 75.25,16.51 75.25,2.22 65.09,2.22
PDI_CLK
  Top 0.305: IC1.35 15.9,53.98 | IC1.35
  Top 0.406: U$1.1 17.78,57.47 17.78,54.93 15.9,53.98
PDI_DATA
  Top 0.305: IC1.34 16.7,47.5 19.05,49.85 22.86,49.85 22.86,57.47 U$1.2
PWMA1
  Top 0.305: J16.1 18.73,28.89 15.9,31.73 IC1.21 | IC1.21 | IC1.21 | J16.1
  Top 0.406: R9.2 J16.1
PWMA2
  Top 0.305: 26.35,26.04 20.32,26.04 15.1,31.25 IC1.20 | IC1.20 | IC1.20
  Top 0.406: 26.35,26.04 R10.2 24.13,26.04 J17.1
PWMB1
  Top 0.305: R14.1 27.07,45.95 25.4,44.28 25.4,41.91 19.82,36.34 IC1.25 | IC1.25
  Top 0.406: J15.1 26.99,46.04 27.07,45.95
PWMB2
  Top 0.305: IC1.24 20.3,35.53 27.3,42.55 R13.1 28.59,44.53 28.59,47.06 29.53,47.77 J14.1 | IC1.24
RX  (1 unrouted)
  Top 0.305: IC1.12 8.7,31.56 8.57,31.43 4.45,26.77 4.45,19.37 8.89,19.37 10.79,21.27
TX  (1 unrouted)
  Top 0.305: 15.24,18.73 15.24,25.08 13.97,26.04 6.99,26.04 6.99,28.26 9.5,31.09 IC1.13
USBDM  (via drill 0.89)
  Top 0.305: X1.D- 10.16,63.98 | 10.16,63.98 10.63,63.98 | IC1.26 18.51,37.15 19.68,37.15 24.05,41.39 24.02,43.71 19.71,48.02 v19.45,48.02 | v13.89,58.66 13.89,61.41 11.3,64.01 10.58,64.01 10.58,64 10.18,64 10.16,63.98
  Bottom 0.305: v19.45,48.02 13.97,53.34 v13.89,58.66
USBDP  (via drill 0.89)
  Top 0.305: IC1.27 19.52,37.94 22.23,40.64 22.23,42.86 v18.1,46.67 | X1.D+ 9.1,63.16 10.58,63.16 12.73,61.01 v12.73,51.72
  Bottom 0.305: v18.1,46.67 v12.73,51.72
V+  (via drill 0.89)
  Top 2.54: T1.2 84.9,62.42 83.57,68.83 C10.+ C9.+ | J3.2 J3.1
  other vias: 71.75,74.61 66.67,74.61 67.94,71.12 78.11,71.12 81.6,66.04 92.39,66.04 81.6,59.37 92.39,59.37 81.28,54.61 88.27,54.61 81.28,46.04 88.27,46.04 88.27,50.16 81.28,50.16 81.6,43.5 92.39,43.5 92.39,49.85 86.68,71.12 84.77,46.04 84.77,50.16 84.77,54.61 87.31,43.5 87,66.04 87,59.37 66.04,83.19 71.44,83.19
  pour Top (rank 2, no thermals): 80.96,64.14 80.96,43.43 93.98,43.43 93.98,64.14
  pour Top: 50.16,73.03 50.16,68.58 80.64,68.58 80.64,64.14 93.98,64.14 93.98,66.1 arc90 86.42,73.66 73.34,73.66 73.34,84.14 65.41,84.14 65.41,73.03
  pour Bottom (rank 2, no thermals): 80.96,64.14 80.96,43.43 93.66,43.43 93.66,64.14
  pour Bottom: 65.41,84.14 65.41,67.94 80.01,67.94 80.64,64.14 93.98,64.14 93.98,66.1 arc90 86.42,73.66 73.34,73.66 73.34,84.14
V_SENSE
  Top 0.305: 33.66,33.33 U5.5 | 33.66,33.33 33.66,34.92 40.32,34.92 | U5.6 33.66,33.33
  Top 0.61: 45.72,34.92 41.91,34.92 40.96,34.92 40.32,34.92 J10.2
  Top 1.27: R8.2 45.72,34.92 R7.1
V_SENSE2
  Top 0.305: U5.10 U5.9 33.66,39.06 33.66,37.47 J10.1
  Top 0.61: J10.1 38.42,37.47 J11.1
VC  (via drill 0.89)
  Top 0.254: U$6.8 61.59,50.8 61.68,50.89 C3.2
  Top 0.305: C3.2 62.99,51.31 63.03,51.22 67.49,51.23 67.92,50.83 | 73.6,47.62 T1.3
  Top 0.61: 67.92,50.83 68.58,50.16
  Top 1.27: T2.2 84.9,20.32 | v66.36,41.91 v78.74,38.1 | C5.+ 51.82,38.89 R7.2 | 68.58,50.16 71.12,47.62 73.6,47.62
  Top 2.54: C5.+ 51.82,38.1 v66.36,38.1 | C6.+ 78.49,38.35 v78.74,38.1 84.9,31.94 84.9,20.32 | v66.36,38.1 62.74,38.1 C7.+ | v66.36,38.1 v66.36,41.91 | C6.+ 73.41,38.1 68.58,38.1 | C6.+ 73.73,38.35 73.73,47.62
  Bottom 2.54: v73.73,45.72 73.74,43.49 73.78,38.18 | 73.78,38.18 75.51,38.33 78.51,38.33 84.14,32.7 | 73.78,38.18 v66.36,41.91 66.04,38.1
  other vias: 81.6,32.7 92.08,32.7 81.92,26.67 92.08,26.67 81.28,22.86 87.95,22.86 87.95,18.73 81.28,18.73 81.28,14.61 87.95,14.61 92.39,19.05 81.92,10.48 92.39,10.79 81.92,4.76 87.31,10.48 86.68,38.1 84.77,14.61 84.77,18.73 84.77,22.86 85.72,4.76 87,26.67 86.68,32.7
  pour Bottom (no thermals): 81.28,33.02 81.28,4.06 93.98,4.06 93.98,33.02
  pour Top (no thermals): 80.96,33.02 80.96,4.06 93.66,4.06 93.66,33.02
  pour Top: 72.39,47.94 arc-45 47.31,40.32 47.31,36.2 80.64,35.88 80.64,33.66 93.66,32.7 arc90 86.36,39.69 76.52,39.69 76.52,47.62
  pour Bottom: 76.52,46.67 76.52,39.69 86.04,39.69 arc-90 93.98,31.75 80.64,31.75 80.64,35.88 62.23,35.88 62.23,40.01 70.48,46.67
VH1
  Top 0.305: U5.4 32.38,28.89
  Top 0.406: R9.1 32.38,28.89 C16.1
VIN
  Top 0.406: U4.5 22.86,76.2 22.86,75.25 22.73,75.25 U4.4
  Top 0.508: JP1.2 22.86,71.62 C14.1
  Top 0.61: 22.73,75.25 C14.1 22.86,71.75
VL1
  Top 0.305: 34.34,30.3 U5.7
  Top 0.406: R10.1 36.2,26.04 36.2,30.48 C15.1 arc-90 34.34,30.3
VOUT1
  Top 0.305: U5.1 30.43,32.38 | 30.43,32.38 30.46,31.6 29.84,31.6 R12.1 | U5.2 31.09,32.38 30.43,32.38 | IC1.22 | 17.14,31.75 16.7,32.2 IC1.22
  Top 0.406: R12.1 arc90 27.15,31.75 22.54,31.75 J19.1 17.14,31.75
VOUT2
  Top 0.305: 27.15,39.37 25.4,39.37 20.8,34.77 20.77,34.73 IC1.23 | IC1.23 | IC1.23 | R11.1 30.48,39.75 | 30.48,39.75 30.92,39.75 31.09,39.58 U5.13 | U5.14 30.43,39.71 30.48,39.75
  Top 0.406: 27.3,40.01 R11.1 arc-90 27.15,39.37 | 20.8,34.77 21.75,34.77 J18.1

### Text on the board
tPlace: REV 1.0 | 12V | V+ | GND | WEDM / PULSE / GENERATOR | WKL 2018 | FAN | + | FAN | + | GND | PULSE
